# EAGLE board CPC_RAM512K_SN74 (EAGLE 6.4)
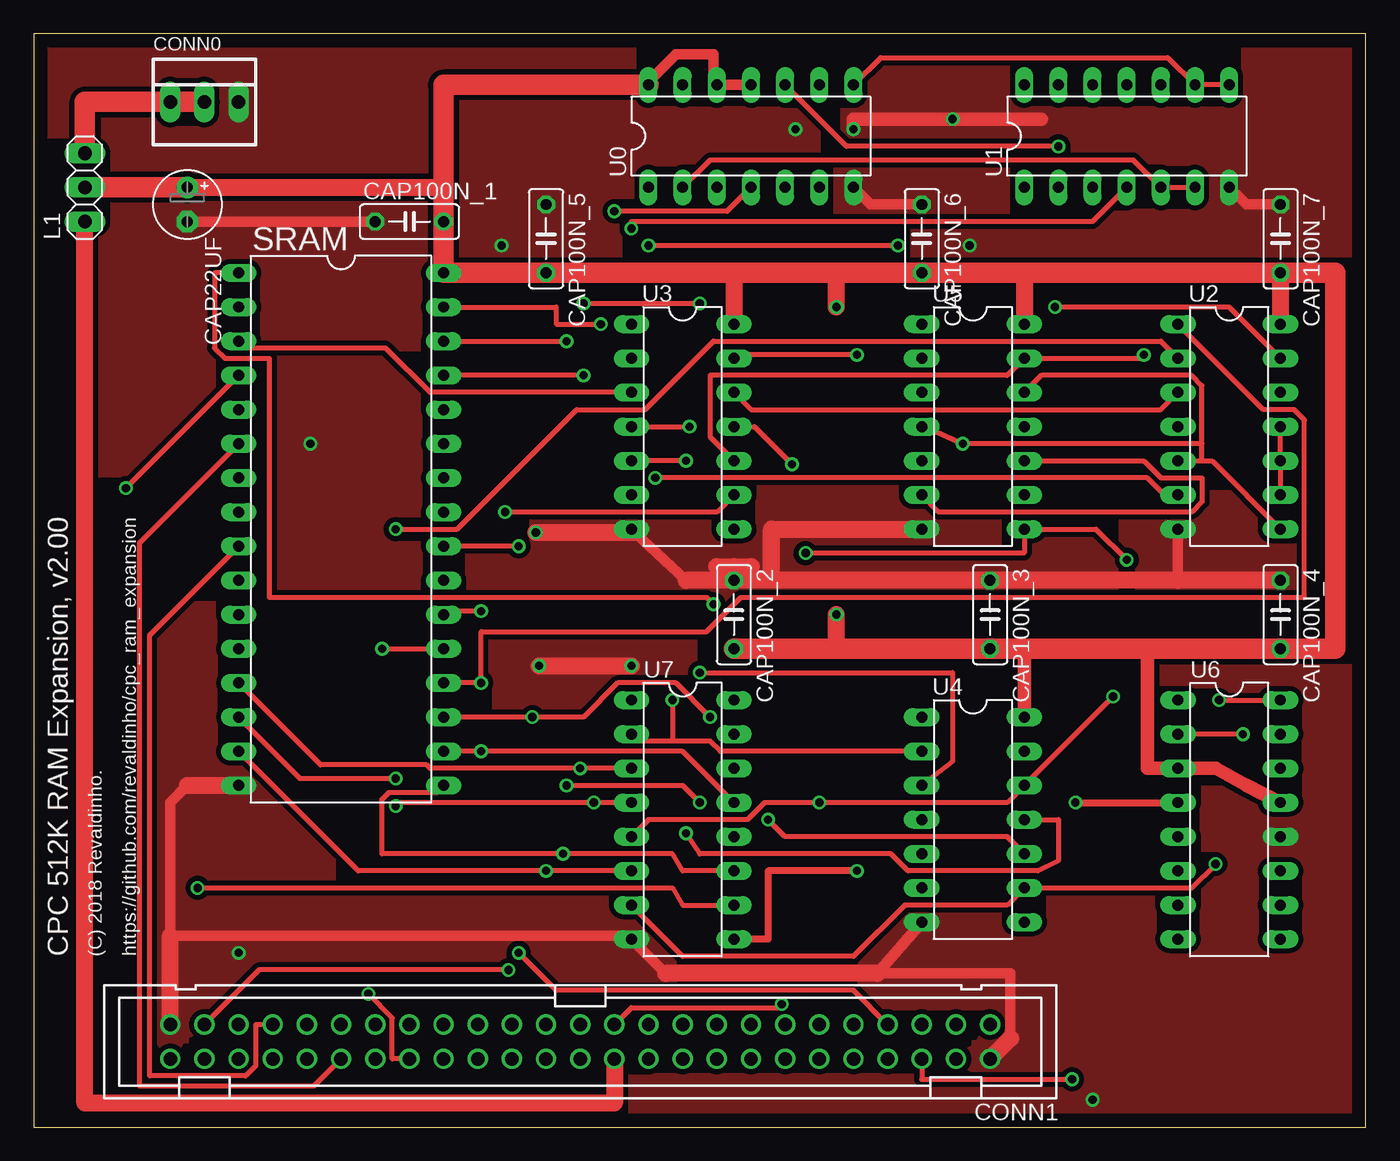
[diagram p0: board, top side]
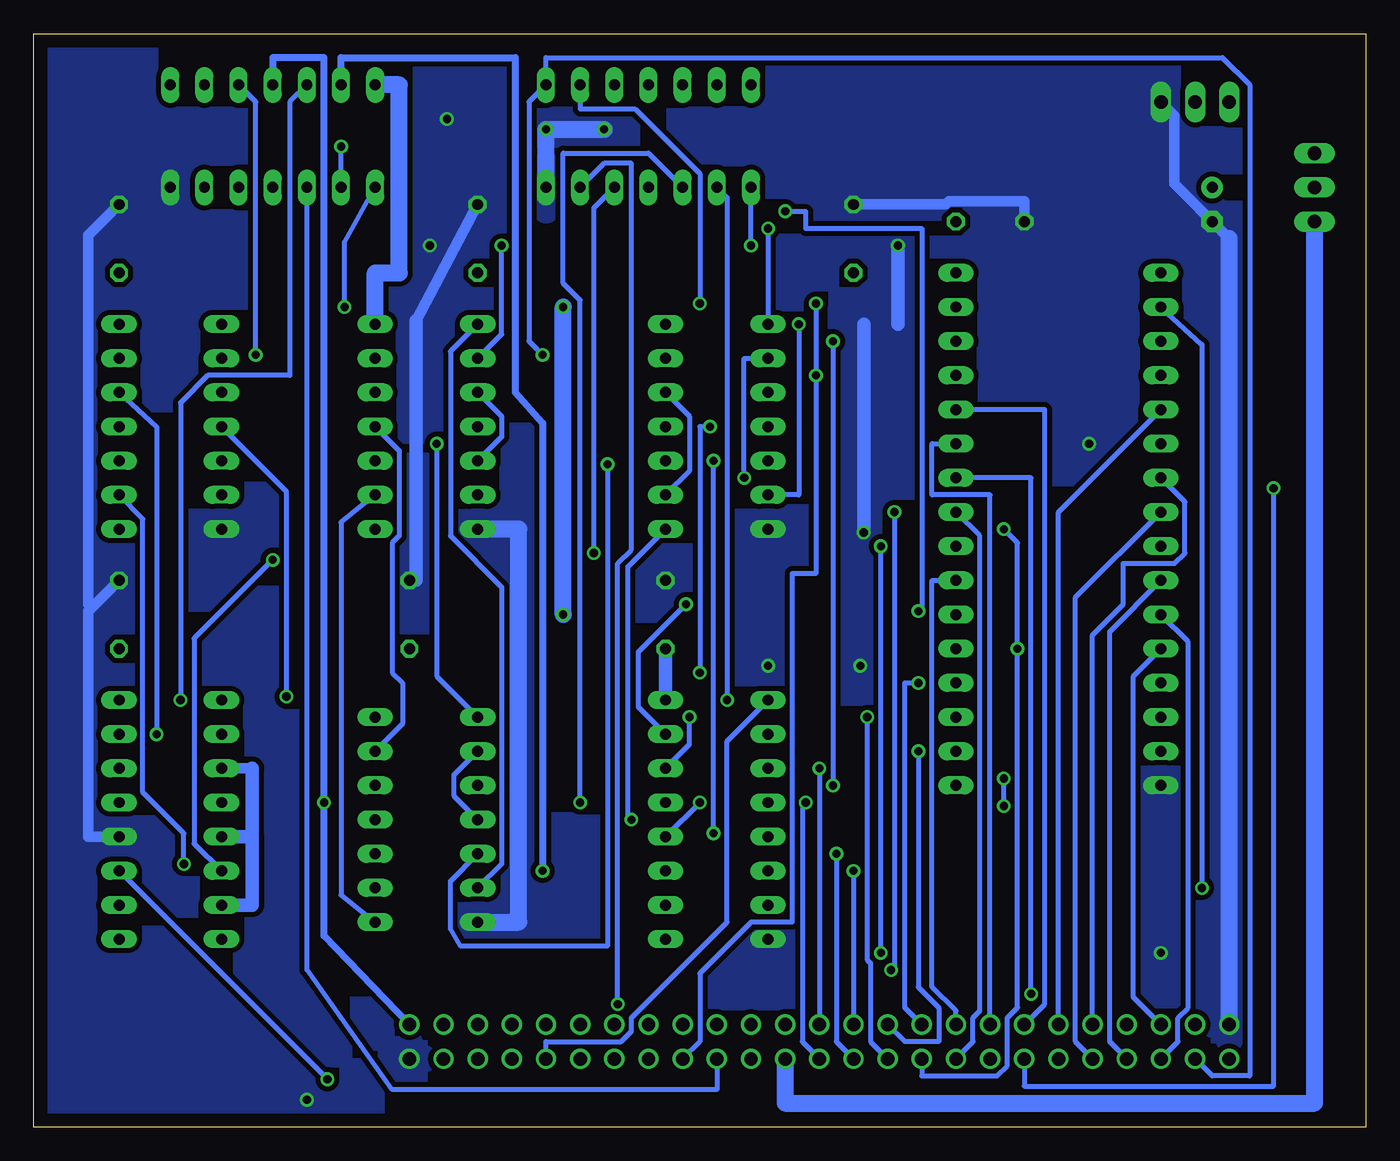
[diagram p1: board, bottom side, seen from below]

Size 99.06 x 81.28 mm. Coordinates in mm from the lower left corner, seen from the top.
Outline: 0,0 99.06,0 99.06,81.28 0,81.28 0,0
Copper layers (1*16): Top 0.035mm / dielectric 1.5mm / Bottom 0.035mm
Design rules "default": minimum track width 10mil, minimum drill 24mil, track to track 8mil, track to pad 8mil, pad to pad 8mil, via to via 8mil, smd to smd 8mil, copper to edge 40mil, drill to drill 8mil, minimum pad ring 10mil, minimum via ring 8mil, stop-mask expansion 4mil, vias tented up to drill 0mil, thermal gap 10mil
Net classes: 0 signal: width 0.356 mm, clearance 0.254 mm; 1 supply: width 0.762 mm, clearance 0.381 mm

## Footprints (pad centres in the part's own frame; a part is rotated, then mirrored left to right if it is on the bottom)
E2,5-5 = drill 0.813 pad 1.6: + -1.27,0 | drill 0.813 pad 1.6 octagon: - 1.27,0
C050-025X075 = drill 0.813 octagon: 1 -2.54,0; 2 2.54,0
22-23-2031 = drill 1 long: 1 -2.54,0; 2 0,0; 3 2.54,0
PAK100/2500-50 = drill 1 pad 1.422: 1 -30.48,-1.27; 2 -30.48,1.27; 3 -27.94,-1.27; 4 -27.94,1.27; 5 -25.4,-1.27; 6 -25.4,1.27; 7 -22.86,-1.27; 8 -22.86,1.27; 9 -20.32,-1.27; 10 -20.32,1.27; 11 -17.78,-1.27; 12 -17.78,1.27; 13 -15.24,-1.27; 14 -15.24,1.27; 15 -12.7,-1.27; 16 -12.7,1.27; 17 -10.16,-1.27; 18 -10.16,1.27; 19 -7.62,-1.27; 20 -7.62,1.27; 21 -5.08,-1.27; 22 -5.08,1.27; 23 -2.54,-1.27; 24 -2.54,1.27; 25 0,-1.27; 26 0,1.27; 27 2.54,-1.27; 28 2.54,1.27; 29 5.08,-1.27; 30 5.08,1.27; 31 7.62,-1.27; 32 7.62,1.27; 33 10.16,-1.27; 34 10.16,1.27; 35 12.7,-1.27; 36 12.7,1.27; 37 15.24,-1.27; 38 15.24,1.27; 39 17.78,-1.27; 40 17.78,1.27; 41 20.32,-1.27; 42 20.32,1.27; 43 22.86,-1.27; 44 22.86,1.27; 45 25.4,-1.27; 46 25.4,1.27; 47 27.94,-1.27; 48 27.94,1.27; 49 30.48,-1.27; 50 30.48,1.27
1X03 = drill 1.016 long: 1 -2.54,0; 2 0,0; 3 2.54,0
DIL32 = drill 0.813 long: 1 -19.05,-7.62; 2 -16.51,-7.62; 3 -13.97,-7.62; 4 -11.43,-7.62; 5 -8.89,-7.62; 6 -6.35,-7.62; 7 -3.81,-7.62; 8 -1.27,-7.62; 9 1.27,-7.62; 10 3.81,-7.62; 11 6.35,-7.62; 12 8.89,-7.62; 13 11.43,-7.62; 14 13.97,-7.62; 15 16.51,-7.62; 16 19.05,-7.62; 17 19.05,7.62; 18 16.51,7.62; 19 13.97,7.62; 20 11.43,7.62; 21 8.89,7.62; 22 6.35,7.62; 23 3.81,7.62; 24 1.27,7.62; 25 -1.27,7.62; 26 -3.81,7.62; 27 -6.35,7.62; 28 -8.89,7.62; 29 -11.43,7.62; 30 -13.97,7.62; 31 -16.51,7.62; 32 -19.05,7.62
DIL14 = drill 0.813 long: 1 -7.62,-3.81; 2 -5.08,-3.81; 3 -2.54,-3.81; 4 0,-3.81; 5 2.54,-3.81; 6 5.08,-3.81; 7 7.62,-3.81; 8 7.62,3.81; 9 5.08,3.81; 10 2.54,3.81; 11 0,3.81; 12 -2.54,3.81; 13 -5.08,3.81; 14 -7.62,3.81
DIL16 = drill 0.813 long: 1 -8.89,-3.81; 2 -6.35,-3.81; 3 -3.81,-3.81; 4 -1.27,-3.81; 5 1.27,-3.81; 6 3.81,-3.81; 7 6.35,-3.81; 8 8.89,-3.81; 9 8.89,3.81; 10 6.35,3.81; 11 3.81,3.81; 12 1.27,3.81; 13 -1.27,3.81; 14 -3.81,3.81; 15 -6.35,3.81; 16 -8.89,3.81

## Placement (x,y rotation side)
CAP22UF  [E2,5-5]  11.43,68.58 270 top
CAP100N_1  [C050-025X075]  27.94,67.31 0 top
CAP100N_2  [C050-025X075]  52.07,38.1 270 top
CAP100N_3  [C050-025X075]  71.12,38.1 270 top
CAP100N_4  [C050-025X075]  92.71,38.1 270 top
CAP100N_5  [C050-025X075]  38.1,66.04 270 top
CAP100N_6  [C050-025X075]  66.04,66.04 270 top
CAP100N_7  [C050-025X075]  92.71,66.04 270 top
CONN0  [22-23-2031]  12.7,76.2 0 top
CONN1  [PAK100/2500-50]  40.64,6.35 180 top
L1  [1X03]  3.81,69.85 90 top
SRAM  [DIL32]  22.86,44.45 270 top
U0  [DIL14]  53.34,73.66 0 top
U1  [DIL14]  81.28,73.66 0 top
U2  [DIL14]  88.9,52.07 270 top
U3  [DIL14]  48.26,52.07 270 top
U4  [DIL14]  69.85,22.86 270 top
U5  [DIL14]  69.85,52.07 270 top
U6  [DIL16]  88.9,22.86 270 top
U7  [DIL16]  48.26,22.86 270 top

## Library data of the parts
CAP22UF CAP100N_1-CAP100N_7 = resistor
CONN0 = con-molex
CONN1 = con-3m
L1 = pinhead
SRAM U0 U1-U7 = ic-package

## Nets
A0: CONN1.33 SRAM.23
A1: CONN1.34 SRAM.25
A2: CONN1.35 SRAM.27
A3: CONN1.36 SRAM.26
A4: CONN1.37 SRAM.28
A5: CONN1.38 SRAM.4
A6: CONN1.39 SRAM.5
A7: CONN1.40 SRAM.6
A8: CONN1.41 SRAM.7
A9: CONN1.42 SRAM.8
A10: CONN1.43 SRAM.9
A11: CONN1.44 SRAM.10
A12: CONN1.45 SRAM.12
A13: CONN1.46 SRAM.11
A14: CONN1.47 U2.3 U3.9 U3.12
A15: CONN1.48 U0.8 U1.8 U1.9 U3.13
BUSACK_B: CONN1.13
BUSRESET_B: CONN1.11
BUSRQ_B: CONN1.14
CLK: CONN1.1 U1.11 U6.4
CLKENB_LAT_Q: U1.12 U6.16
CURSOR: CONN1.5
D0: CONN1.25 SRAM.13 U7.3
D1: CONN1.26 SRAM.14 U7.4
D2: CONN1.27 SRAM.15 U7.6
D3: CONN1.28 SRAM.17 U7.11
D4: CONN1.29 SRAM.18 U7.13
D5: CONN1.30 SRAM.19 U7.14
D6: CONN1.31 SRAM.20 U2.1
D7: CONN1.32 SRAM.21 U2.2
EXP_B: CONN1.3
EXTRAM_B: U0.5 U5.8 U6.6
HALT_B: CONN1.17
INT_B: CONN1.16
IOREQ_B: CONN1.20 U1.3
LPEN: CONN1.4
M1_B: CONN1.22
MREQ_B: CONN1.23 U0.6
N14: U2.12 U6.2
N15: U1.1 U2.13
N16: U2.6 U3.2
N17: U1.4 U3.1
N18: U4.13 U5.11
N19: U3.5 U4.11
N20: U3.4 U4.3
N21: U1.10 U3.10 U5.13
N22: U3.8 U4.10
N23: U3.11 U4.5
N24: U0.1 U5.2
N25: U4.6 U5.1
N26: U5.3 U5.5
N27: U2.5 U2.8 U4.1 U5.4 U5.12
N28: U5.6 U5.10
N29: U4.8 U5.9
NMI_B: CONN1.15
NN1: U0.10 U1.2
RAMADRHI0: SRAM.3 U3.3
RAMADRHI1: SRAM.31 U3.6
RAMADRHI2: SRAM.2 U7.10
RAMADRHI3: SRAM.30 U7.12
RAMADRHI4: SRAM.1 U7.15
RAMBLOCK_Q0: U0.2 U1.5 U1.6 U4.2 U4.4 U7.2
RAMBLOCK_Q1: U0.3 U2.4 U4.12 U7.5
RAMBLOCK_Q2: U2.9 U2.10 U2.11 U4.9 U7.7
RAMCS_B: SRAM.22 U0.4
RAMDIS: CONN1.6 U6.11
RAMRD_B: CONN1.7 SRAM.24
RD_B: CONN1.19
READY: CONN1.12
RESET_B: CONN1.10 U7.1
RFSH_B: CONN1.21
ROMDIS: CONN1.8
ROMEN_B: CONN1.9
SOUND: CONN1.50
VDD [supply]: CAP22UF.+ CAP100N_1.2 CAP100N_2.2 CAP100N_3.2 CAP100N_4.2 CAP100N_5.2 CAP100N_6.2 CAP100N_7.2 L1.2 SRAM.32 U0.11 U0.12 U0.14 U1.14 U2.14 U3.14 U4.14 U5.14 U6.3 U6.5 U6.7 U6.13 U7.16
VDD_CPC [supply]: CONN1.24 L1.1
VDD_EXT [supply]: CONN0.1 CONN0.2 L1.3
VSS [supply]: CAP22UF.- CAP100N_1.1 CAP100N_2.1 CAP100N_3.1 CAP100N_4.1 CAP100N_5.1 CAP100N_6.1 CAP100N_7.1 CONN0.3 CONN1.2 CONN1.49 SRAM.16 U0.7 U1.7 U2.7 U3.7 U4.7 U5.7 U6.12 U7.8
WCLK_B: U1.13 U7.9
WR_B: CONN1.18 SRAM.29 U0.9

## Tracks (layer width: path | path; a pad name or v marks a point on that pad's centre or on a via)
A0
  Bottom 0.356: SRAM.23 32.26,40.64 32.26,10.41 30.48,8.64 CONN1.33
A1
  Bottom 0.356: SRAM.25 28.7,43.94 28.7,8.64 29.21,8.13 29.21,6.35 CONN1.34
A2
  Bottom 0.356: SRAM.27 32.26,50.8 32.26,46.99 27.94,46.99 CONN1.35
A3  (via drill 0.61)
  Top 0.356: v24.89,9.91 26.67,8.13 26.67,5.08 CONN1.36
  Bottom 0.356: SRAM.26 24.89,48.26 v24.89,9.91
A4
  Bottom 0.356: SRAM.28 23.88,53.34 23.88,9.14 CONN1.37
A5  (via drill 0.61)
  Top 0.356: v6.86,47.5 SRAM.4
  Bottom 0.356: v6.86,47.5 6.86,3.05 25.4,3.05 CONN1.38
A6
  Bottom 0.356: SRAM.5 22.86,45.72 CONN1.39
A7
  Top 0.356: SRAM.6 7.87,43.43 7.87,3.05 20.83,3.05 CONN1.40
A8
  Bottom 0.356: SRAM.7 13.46,46.48 13.46,42.67 14.22,41.91 18.03,41.91 18.03,38.86 20.32,36.58 CONN1.41
A9
  Bottom 0.356: SRAM.8 21.59,39.37 21.59,6.35 CONN1.42
A10
  Top 0.356: SRAM.9 8.64,36.58 8.64,3.81 15.75,3.81 16.51,4.57 16.51,7.62 CONN1.43
A11
  Bottom 0.356: SRAM.10 19.05,36.83 19.05,6.35 CONN1.44
A12
  Bottom 0.356: SRAM.12 17.27,33.53 17.27,9.65 CONN1.45
A13
  Bottom 0.356: SRAM.11 13.21,36.07 13.21,8.89 13.97,8.13 13.97,6.35 CONN1.46
A14  (via drill 0.61)
  Top 0.356: U2.3 83.82,53.34 53.34,53.34 U3.12 | CONN1.47 16.76,11.68 v35.31,11.68 | v35.05,45.72 50.8,45.72 U3.9
  Bottom 0.356: U3.9 50.29,48.77 50.29,52.83 U3.12 | v35.31,11.68 35.05,11.94 v35.05,45.72
A15  (via drill 0.61)
  Top 0.356: U1.8 U1.9 84.33,79.5 62.99,79.5 U0.8 | U3.13 52.32,57.4 v61.21,57.4
  Bottom 0.356: v61.21,57.4 62.23,58.42 62.23,76.2 U0.8 60.96,79.5 10.67,79.5 8.64,77.47 8.64,3.81 11.43,3.81 CONN1.48
CLK  (via drill 0.61)
  Top 0.508: v77.47,24.13 U6.4
  Bottom 0.508: CONN1.1 77.47,14.22 v77.47,24.13 77.47,79.5 81.28,79.5 U1.11
CLKENB_LAT_Q  (via drill 0.61)
  Top 0.356: v88.14,31.75 U6.16
  Bottom 0.356: v88.14,31.75 88.14,53.85 86.11,55.88 80.01,55.88 80.01,76.2 U1.12
D0  (via drill 0.61)
  Top 0.356: SRAM.13 21.34,26.92 29.21,26.92 29.46,26.67 v40.64,26.67 U7.3
  Bottom 0.356: v40.64,26.67 CONN1.25
D1  (via drill 0.61)
  Top 0.356: SRAM.14 19.81,25.91 v26.92,25.91 | v26.92,23.88 27.18,24.13 v41.66,24.13 U7.4
  Bottom 0.356: v26.92,23.88 v26.92,25.91 | CONN1.26 41.91,6.35 41.91,23.88 v41.66,24.13
D2  (via drill 0.61)
  Top 0.356: SRAM.15 24.13,19.05 v38.1,19.05 U7.6
  Bottom 0.356: v38.1,19.05 CONN1.27
D3  (via drill 0.61)
  Top 0.356: SRAM.17 29.97,24.89 26.42,24.89 25.91,24.38 25.91,20.32 v39.37,20.32 47.5,20.32 48.26,19.05 U7.11
  Bottom 0.356: CONN1.28 39.37,6.35 v39.37,20.32
D4  (via drill 0.61)
  Top 0.356: SRAM.18 v33.27,27.94 48.26,27.94 U7.13
  Bottom 0.356: CONN1.29 34.29,6.35 31.75,6.35 31.75,8.89 33.27,10.41 v33.27,27.94
D5  (via drill 0.61)
  Top 0.356: SRAM.19 v37.08,30.48 40.89,30.48 43.43,33.02 47.75,33.02 v50.29,30.48
  Bottom 0.356: v50.29,30.48 50.29,28.45 U7.14 | CONN1.30 36.83,6.35 36.83,12.19 37.08,12.45 v37.08,30.48
D6  (via drill 0.61)
  Top 0.356: v33.27,33.02 SRAM.20 | v33.27,33.02 33.53,33.02 | U2.1 91.44,53.34 93.73,53.34 94.49,52.58 94.49,39.37 52.58,39.37 50.04,36.83 33.27,36.83 v33.27,33.02
  Bottom 0.356: v33.27,33.02 34.29,33.02 34.29,8.89 CONN1.31
D7  (via drill 0.61)
  Top 0.356: v25.91,35.56 SRAM.21 | U2.2 83.82,58.42 50.55,58.42 45.47,53.34 40.39,53.34 31.5,44.45 v26.92,44.45
  Bottom 0.356: CONN1.32 33.02,3.81 27.43,3.81 26.67,4.57 26.67,8.13 25.91,8.89 v25.91,35.56 25.91,43.43 v26.92,44.45
EXTRAM_B  (via drill 0.61)
  Top 0.356: v81.28,42.16 78.99,44.45 U5.8 73.66,42.67 v57.4,42.67
  Bottom 0.356: U6.6 87.12,21.08 87.12,36.32 v81.28,42.16 | U0.5 57.4,68.33 v57.4,42.67
IOREQ_B
  Bottom 0.356: U1.3 78.74,11.68 72.39,2.79 48.26,2.79 CONN1.20
MREQ_B  (via drill 0.61)
  Top 0.356: v55.63,9.14 55.37,8.89 44.45,8.89 CONN1.23
  Bottom 0.356: U0.6 56.64,71.63 54.61,71.63 54.61,42.93 55.63,41.91 v55.63,9.14
N14  (via drill 0.61)
  Top 0.356: v89.92,29.21 U6.2
  Bottom 0.356: v89.92,29.21 89.92,52.07 U2.12
N15  (via drill 0.61)
  Top 0.356: v75.95,60.96 88.9,60.96 U2.13
  Bottom 0.356: U1.1 75.95,65.79 v75.95,60.96
N16  (via drill 0.61)
  Top 0.356: v46.23,48.26 82.8,48.26 84.07,46.99 U2.6
  Bottom 0.356: U3.2 46.23,57.15 v46.23,48.26
N17  (via drill 0.61)
  Top 0.356: v44.45,66.8 44.45,67.31 78.74,67.31 U1.4
  Bottom 0.356: v44.45,66.8 U3.1
N18
  Bottom 0.356: U4.13 71.63,29.97 71.63,33.02 72.39,33.78 72.39,43.43 71.88,43.94 71.88,50.29 U5.11
N19  (via drill 0.61)
  Top 0.356: v48.51,49.53 U3.5 | v48.51,21.84 49.53,20.32 63.75,20.32 65.02,19.05 74.68,19.05 76.2,19.81 76.2,22.86 U4.11
  Bottom 0.356: v48.51,21.84 v48.51,49.53
N20  (via drill 0.61)
  Top 0.356: U4.3 68.33,27.18 68.33,33.78 v49.53,33.78 | U3.4 v48.77,52.07
  Bottom 0.356: v49.53,33.78 49.53,52.07 v48.77,52.07
N21  (via drill 0.61)
  Top 0.356: U3.10 50.29,51.31 50.29,55.88 72.39,55.88 U5.13 82.3,57.15 v82.55,57.4
  Bottom 0.356: U1.10 82.55,76.2 v82.55,57.4
N22  (via drill 0.61)
  Top 0.356: v54.61,22.86 55.88,21.59 72.39,21.59 U4.10
  Bottom 0.356: U3.8 54.86,41.66 54.86,23.11 v54.61,22.86
N23  (via drill 0.61)
  Top 0.356: v56.39,49.28 53.59,52.07 U3.11
  Bottom 0.356: U4.5 68.07,18.29 68.07,14.73 67.31,13.46 56.39,13.46 v56.39,49.28
N24  (via drill 0.61)
  Top 0.356: v64.26,65.53 v45.72,65.53
  Bottom 0.356: v45.72,65.53 U0.1 | v64.26,65.53 64.26,58.93 U5.2
N25
  Bottom 0.356: U4.6 64.26,19.56 64.26,40.13 68.07,43.94 68.07,57.66 U5.1
N26
  Bottom 0.356: U5.5 64.26,51.31 64.26,52.83 U5.3
N27  (via drill 0.61)
  Top 0.356: U5.4 66.29,52.07 v69.09,50.8 86.87,50.8 | U5.12 74.93,55.88 86.11,55.88 86.87,55.12 86.87,50.8 | 86.87,49.53 86.87,50.8 | U2.5 86.87,49.53 | U2.8 87.63,49.53 86.87,49.53
  Bottom 0.356: U4.1 69.09,33.53 v69.09,50.8
N28
  Top 0.356: U5.6 67.31,45.72 86.11,45.72 86.87,46.48 86.87,48.26 83.82,48.26 82.55,49.53 U5.10
N29
  Bottom 0.356: U4.8 76.2,17.27 76.2,44.96 U5.9
NN1  (via drill 0.61)
  Top 0.356: U0.10 60.45,72.9 v76.2,72.9
  Bottom 0.356: U1.2 v76.2,72.9
RAMADRHI0
  Top 0.356: SRAM.3 15.75,57.91 26.16,57.91 29.46,54.61 U3.3
RAMADRHI1  (via drill 0.61)
  Top 0.356: SRAM.31 38.86,60.96 38.86,59.69 v42.16,59.69
  Bottom 0.356: U3.6 42.16,46.99 v42.16,59.69
RAMADRHI2  (via drill 0.61)
  Top 0.356: U7.10 48.26,16.51 47.5,17.78 v12.19,17.78
  Bottom 0.356: v12.19,17.78 12.19,58.17 SRAM.2
RAMADRHI3  (via drill 0.61)
  Top 0.356: v49.53,24.13 48.26,25.4 v39.62,25.4 | SRAM.30 v39.62,58.42
  Bottom 0.356: v49.53,24.13 U7.12 | v39.62,58.42 v39.62,25.4
RAMADRHI4  (via drill 0.61)
  Top 0.356: v50.55,38.86 50.04,39.37 17.53,39.37 17.53,57.15 14.22,57.15 13.46,57.91 13.46,63.5 SRAM.1
  Bottom 0.356: U7.15 54.1,31.24 54.1,35.31 v50.55,38.86
RAMBLOCK_Q0  (via drill 0.61)
  Top 0.356: U7.2 44.96,28.7 47.5,28.7 | 47.5,28.7 50.29,28.7 51.05,27.94 U4.2 | U0.2 50.29,71.88 81.79,71.88 U1.5 U1.6 | v47.5,31.75 47.5,28.7
  Bottom 0.356: U4.4 67.82,24.64 67.82,26.16 U4.2 | v47.5,31.75 47.5,69.09 U0.2
RAMBLOCK_Q1  (via drill 0.61)
  Top 0.356: U7.5 45.72,22.86 53.09,22.86 54.36,24.13 v58.42,24.13 72.39,24.13 U4.12 v80.26,32
  Bottom 0.356: U0.3 53.34,72.39 59.69,72.39 59.69,62.74 58.42,61.47 v58.42,24.13 | U2.4 80.26,47.24 v80.26,32
RAMBLOCK_Q2  (via drill 0.61)
  Top 0.356: U2.9 U2.10 U2.11 | U7.7 48.26,12.7 60.96,12.7 64.77,16.51 72.39,16.51 U4.9 86.11,17.78 v87.88,19.56
  Bottom 0.356: U2.9 90.93,45.21 90.93,24.89 87.88,21.84 v87.88,19.56
RAMCS_B  (via drill 0.61)
  Top 0.356: SRAM.22 30.73,38.35 v33.27,38.35 | v43.18,68.07 51.56,68.07 U0.4
  Bottom 0.356: v33.27,38.35 33.02,38.61 33.02,66.8 41.66,66.8 41.66,68.07 v43.18,68.07
RAMDIS  (via drill 0.61)
  Top 0.356: v77.22,3.56 66.04,3.56 CONN1.6
  Bottom 0.356: v77.22,3.56 U6.11
RAMRD_B  (via drill 0.61)
  Top 0.356: v36.07,43.18 SRAM.24 | v36.07,12.95 38.86,10.16 60.96,10.16 CONN1.7
  Bottom 0.356: v36.07,12.95 v36.07,43.18
RESET_B
  Bottom 0.356: U7.1 47.5,28.7 47.5,15.24 54.61,8.13 54.61,7.11 55.37,6.35 60.96,6.35 CONN1.10
VDD  (via drill 0.61)
  Top 0.762: U0.11 U0.12 50.55,77.72 50.55,79.76 47.75,79.76 45.97,77.98 U0.14
  Top 1.016: U6.13 90.17,25.4 87.88,26.67 U6.3 82.8,26.67 82.8,35.56 | 73.66,35.56 U4.14
  Top 1.27: CAP22UF.+ 30.48,69.85 CAP100N_1.2 | v59.69,60.96 59.69,63.5 | 59.69,35.56 v59.69,38.1 | 52.07,63.5 U3.14 | 73.66,63.5 U5.14 | CAP100N_7.2 U2.14
  Top 1.524: CAP100N_2.2 59.69,35.56 CAP100N_3.2 73.66,35.56 82.8,35.56 CAP100N_4.2 96.77,35.56 96.77,63.5 CAP100N_7.2 73.66,63.5 CAP100N_6.2 59.69,63.5 52.07,63.5 CAP100N_5.2 SRAM.32 CAP100N_1.2 30.48,77.47 U0.14 | CAP22UF.+ L1.2
  Bottom 0.762: 82.8,26.67 U6.3
  Bottom 1.016: U6.7 82.8,16.51 82.8,21.59 | U6.5 82.8,21.59 | 82.8,21.59 82.8,26.67 | CAP100N_2.2 U7.16
  Bottom 1.27: v59.69,38.1 v59.69,60.96 | U1.14 71.88,77.47 71.88,63.5 73.66,63.5 U5.14
VDD_CPC
  Top 1.27: CONN1.24 43.18,1.78 3.81,1.78 L1.1
  Bottom 1.27: CONN1.24 43.18,1.78 3.81,1.78 L1.1
VDD_EXT
  Top 1.524: L1.3 3.81,76.2 CONN0.1 CONN0.2
  Bottom 1.27: CONN0.2 12.7,76.45
VSS  (via drill 0.61)
  Top 0.762: U0.7 62.23,68.58 CAP100N_6.1 | U1.7 90.17,68.58 CAP100N_7.1 | 48.51,40.64 44.7,44.2 U3.7 | 85.09,40.64 U2.7 | CAP22UF.- CAP100N_1.1 | 11.43,25.4 10.16,24.13 10.16,14.22 44.2,14.22 U7.8 46.99,11.43 | U4.7 62.74,11.43 72.64,11.43 72.64,6.6 | 52.07,41.66 CAP100N_2.1
  Top 1.016: 74.93,74.93 v68.33,74.93 60.96,74.93 v60.96,74.17
  Top 1.27: CAP100N_4.1 85.09,40.64 CAP100N_3.1 CAP100N_2.1 48.51,40.64 | U5.7 54.86,44.45 54.86,41.15 | 11.43,25.4 SRAM.16 | CONN1.49 10.16,14.22 | 62.74,11.43 46.99,11.43 | 72.64,6.6 CONN1.2 | 44.7,44.2 v37.34,44.2 | v37.59,34.29 v44.45,34.29 | 50.8,41.66 52.07,41.66 53.34,41.66
  Bottom 0.762: U6.12 95,21.59 95,38.35 94.74,38.61 | CAP100N_4.1 94.74,38.61 | CAP100N_7.1 95,66.29 95,38.86 94.74,38.61 | 70.61,59.94 CAP100N_6.1 | CAP100N_3.1 70.61,40.64 | CAP100N_5.1 31.24,68.58 30.99,68.83 25.4,68.83 CAP100N_1.1 | CONN0.3 14.22,75.18 14.22,70.1 CAP22UF.- 10.16,66.04 | v56.64,74.17 56.39,74.17
  Bottom 1.016: 70.61,40.64 70.61,59.94 | v37.34,44.2 37.34,59.69 | 34.8,59.69 v34.8,65.53
  Bottom 1.27: CONN1.49 10.16,66.04 | U5.7 62.99,44.45 62.99,15.24 U4.7 | U0.7 v60.96,74.17 v56.64,74.17
  other vias: 69.6,65.53 78.74,2.03 20.57,50.8 15.24,12.95
  pour Top: 0,0 0,81.28 99.06,81.28 99.06,0
  pour Bottom: 0,0 0,81.28 99.06,81.28 99.06,0
WCLK_B  (via drill 0.61)
  Top 0.508: U7.9 54.61,13.97 54.61,19.05 v61.21,19.05
  Bottom 0.508: v61.21,19.05 61.21,52.32 63.25,54.61 63.25,79.5 76.2,79.5 U1.13
WR_B  (via drill 0.61)
  Top 0.356: v40.89,55.88 SRAM.29 | v49.53,61.21 v40.89,61.21
  Bottom 0.356: v40.89,61.21 v40.89,55.88 40.89,41.15 42.67,41.15 42.67,15.24 45.72,15.24 49.53,11.43 49.53,6.35 CONN1.18 | v49.53,61.21 49.53,70.87 54.36,75.69 58.42,75.69 U0.9

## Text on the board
tPlace: CPC 512K RAM Expansion, v2.00 | (C) 2018 Revaldinho. | https://github.com/revaldinho/cpc_ram_expansion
